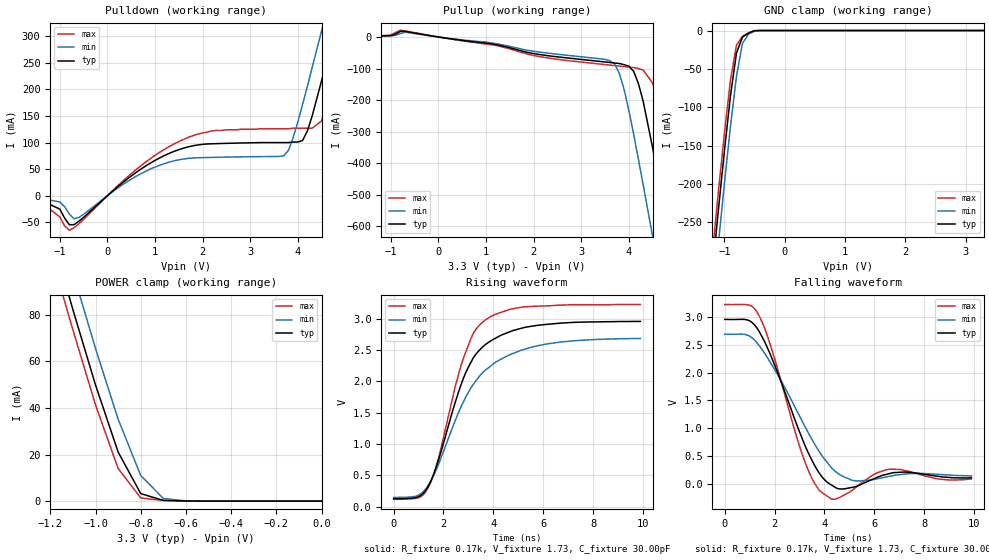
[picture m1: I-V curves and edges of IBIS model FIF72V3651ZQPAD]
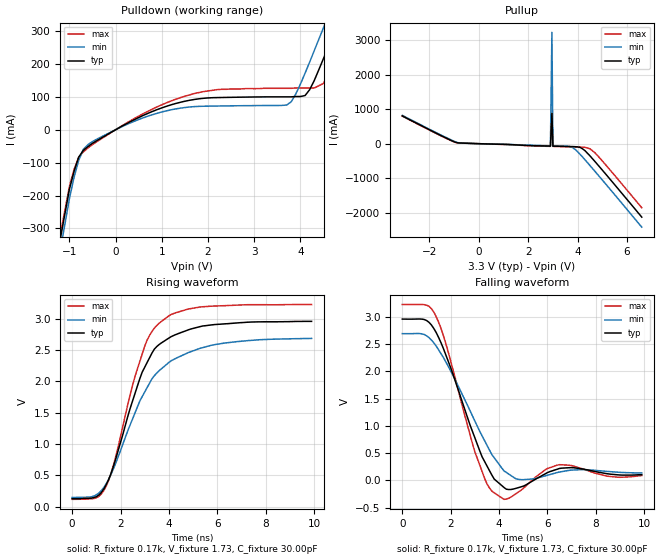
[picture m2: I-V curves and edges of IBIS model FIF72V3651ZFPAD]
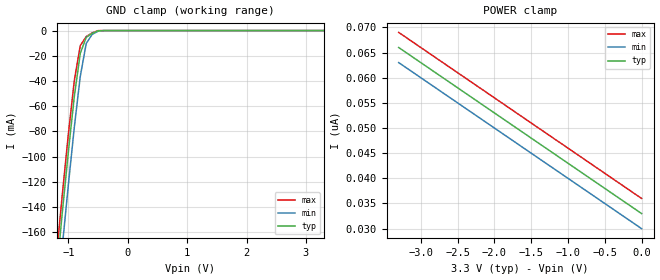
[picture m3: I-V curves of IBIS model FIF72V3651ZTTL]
| IBIS file i72v3641.ibs created by s2ibis2 version 1.1
| North Carolina State University Electronics Research Laboratory  1995
[IBIS ver]   2.1
[File name]   i72v3641.ibs
[File Rev]   1.0
[Date]   05/01/98
[Source]   Integrated Device Technology, Inc.
[Notes]   1. Temperatures: typ=25C, min=70C, max=0C 2. Cemos8_3.3v
   process. 3. Ramp rates based on 50 ohm load.
[Copyright]   Copyright 1997, Integrated Device Technology, Inc.
|   Component idt72V3641
[Component]   idt72V3641
[Manufacturer]   Integrated Device Technology
[Package]
| variable   typ   min   max
R_pkg   0.75   0.60   0.90
L_pkg   8.10nH   8.30nH   9.90nH
C_pkg   0.53pF   0.46pF   0.60pF
[Pin]  signal_name   model_name   R_pin   L_pin   C_pin
1   A35   FIF72V3651ZQPAD
2   A34   FIF72V3651ZQPAD
3   A33   FIF72V3651ZQPAD
4   A32   FIF72V3651ZQPAD
5   VCC   POWER
6   A31   FIF72V3651ZQPAD
7   A30   FIF72V3651ZQPAD
8   GND   GND
9   A29   FIF72V3651ZQPAD
10   A28   FIF72V3651ZQPAD
11   A27   FIF72V3651ZQPAD
12   A26   FIF72V3651ZQPAD
13   A25   FIF72V3651ZQPAD
14   A24   FIF72V3651ZQPAD
15   A23   FIF72V3651ZQPAD
16   GND   GND
17   A22   FIF72V3651ZQPAD
18   VCC   POWER
19   A21   FIF72V3651ZQPAD
20   A20   FIF72V3651ZQPAD
21   A19   FIF72V3651ZQPAD
22   A18   FIF72V3651ZQPAD
23   GND   GND
24   A17   FIF72V3651ZQPAD
25   A16   FIF72V3651ZQPAD
26   A15   FIF72V3651ZQPAD
27   A14   FIF72V3651ZQPAD
28   A13   FIF72V3651ZQPAD
29   VCC   POWER
30   A12   FIF72V3651ZQPAD
31   GND   GND
32   A11   FIF72V3651ZQPAD
33   A10   FIF72V3651ZQPAD
34   A9   FIF72V3651ZQPAD
35   A8   FIF72V3651ZQPAD
36   A7   FIF72V3651ZQPAD
37   A6   FIF72V3651ZQPAD
38   GND   GND
39   A5   FIF72V3651ZQPAD
40   A4   FIF72V3651ZQPAD
41   A3   FIF72V3651ZQPAD
42   VCC   POWER
43   A2   FIF72V3651ZQPAD
44   A1   FIF72V3651ZQPAD
45   A0   FIF72V3651ZQPAD
46   GND   GND
47   B0   FIF72V3651ZQPAD
48   B1   FIF72V3651ZQPAD
49   B2   FIF72V3651ZQPAD
50   B3   FIF72V3651ZQPAD
51   B4   FIF72V3651ZQPAD
52   A5   FIF72V3651ZQPAD
53   GND   GND
54   B6   FIF72V3651ZQPAD
55   VCC   POWER
56   B7   FIF72V3651ZQPAD
57   B8   FIF72V3651ZQPAD
58   B9   FIF72V3651ZQPAD
59   B10   FIF72V3651ZQPAD
60   B11   FIF72V3651ZQPAD
61   GND   GND
62   B12   FIF72V3651ZQPAD
63   B13   FIF72V3651ZQPAD
64   B14   FIF72V3651ZQPAD
65   B15   FIF72V3651ZQPAD
66   VCC   POWER
67   B16   FIF72V3651ZQPAD
68   B17   FIF72V3651ZQPAD
69   GND   GND
70   B18   FIF72V3651ZQPAD
71   B19   FIF72V3651ZQPAD
72   B20   FIF72V3651ZQPAD
73   B21   FIF72V3651ZQPAD
74   B22   FIF72V3651ZQPAD
75   B23   FIF72V3651ZQPAD
76   GND   GND
77   B24   FIF72V3651ZQPAD
78   B25   FIF72V3651ZQPAD
79   VCC   POWER
80   B26   FIF72V3651ZQPAD
81   B27   FIF72V3651ZQPAD
82   B28   FIF72V3651ZQPAD
83   B29   FIF72V3651ZQPAD
84   B30   FIF72V3651ZQPAD
85   B31   FIF72V3651ZQPAD
86   GND   GND
87   B32   FIF72V3651ZQPAD
88   B33   FIF72V3651ZQPAD
89   B34   FIF72V3651ZQPAD
90   B35   FIF72V3651ZQPAD
91   VCC   POWER
92   CLKB   FIF72V3651ZTTL
93   ENB   FIF72V3651ZTTL
94   WLRB   FIF72V3651ZTTL
95   CSBL   FIF72V3651ZTTL
96   GND   GND
97   MBF1L   FIF72V3651ZFPAD
98   GND   GND
99   MBB   FIF72V3651ZTTL
100   NC   NC
101   VCC   POWER
102   RFM   FIF72V3651ZTTL
103   RTM   FIF72V3651ZTTL
104   FS1SENL   FIF72V3651ZTTL
105   FS0SD   FIF72V3651ZTTL
106   GND   GND
107   RSTL   FIF72V3651ZTTL
108   MBA   FIF72V3651ZTTL
109   MBF2L   FIF72V3651ZFPAD
110   VCC   POWER
111   AEL   FIF72V3651ZFPAD
112   AFL   FIF72V3651ZFPAD
114   OR   FIF72V3651ZFPAD
115   IR   FIF72V3651ZFPAD
116   CSAL   FIF72V3651ZTTL
117   WRLA   FIF72V3651ZTTL
118   ENA   FIF72V3651ZTTL
119   CLKA   FIF72V3651ZTTL
120   GND   GND
| Models and submodels in the file (3): FIF72V3651ZQPAD (I/O), FIF72V3651ZFPAD (Output), FIF72V3651ZTTL (Input)
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| FIN  FIN   dummy_model
| QIN  QIN   dummy_model
| QOEL QOEL   dummy_model
|   Model FIF72V3651ZQPAD
[Model]   FIF72V3651ZQPAD
Model_type   I/O
Polarity   Non-Inverting
Enable   Active-Low
Vinl =  0.800V
Vinh =  2.000V
Vmeas =  1.500V
C_comp   3.00pF   NA   NA
[Temperature Range]   25.00   70.00   0.000
[Voltage Range]   3.30V   3.00V   3.60V
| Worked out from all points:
|   slope of the pulldown table from 0 to 0.495 V, typ, clamps not added: 13.5 ohm
|   slope of the pullup table from 0 to 0.495 V, typ, clamps not added: 46.5 ohm
|   GND clamp passes 1 mA (typ) near -0.52 V on its own axis
|   POWER clamp passes 1 mA (typ) near -0.72 V on its own axis
|   rising waveform, R_fixture 0.17k, V_fixture 1.73, C_fixture 30.00pF: 20-80 % time 1.47ns typ, 1.9ns min, 1.25ns max; typ from 0.128 V to 2.96 V
|   falling waveform, R_fixture 0.17k, V_fixture 1.73, C_fixture 30.00pF: 20-80 % time 1.46ns typ, 1.86ns min, 1.22ns max; typ from 2.96 V to 0.105 V
[Pulldown]
| voltage   I(typ)   I(min)   I(max)
-3.3V     -1mA       -1mA       -1mA
-1.5V     -4.2mA     -3.2mA     -5mA
-800mV    -54.6mA    -34.52mA   -64.94mA
-600mV    -47.99mA   -40.8mA    -52.81mA
600mV     43.67mA    36.44mA    48.95mA
1.5V      86.71mA    67.57mA    102mA
3.7V      100mA      75.02mA    126mA
4.1V      104mA      172mA      127mA
4.5V      217mA      311mA      141mA
4.7V      287mA      383mA      200mA
5.1V      430mA      528mA      340mA
6.6V      980mA      1.077A     888mA
[Pullup]
| voltage   I(typ)   I(min)   I(max)
-3.3V     300uA      300uA      300uA
-800mV    17.75mA    10.87mA    21.29mA
3.6V      -80.87mA   -75.44mA   -89.18mA
3.9V      -87.82mA   -167mA     -93.93mA
4.1V      -109mA     -309mA     -97.12mA
4.3V      -204mA     -469mA     -105mA
4.5V      -353mA     -634mA     -147mA
4.7V      -515mA     -801mA     -262mA
4.9V      -682mA     -970mA     -418mA
5.1V      -851mA     -1.14A     -583mA
5.3V      -1.02A     -1.31A     -751mA
6.6V      -2.136A    -2.428A    -1.864A
[GND_clamp]
| voltage   I(typ)   I(min)   I(max)
-3.3V     -2.102A    -2.142A    -2.08A
-1.2V     -314mA     -358mA     -291mA
-1.1V     -234mA     -278mA     -210mA
-1V       -157mA     -199mA     -134mA
-900mV    -85.1mA    -125mA     -64.47mA
-800mV    -29.4mA    -59.48mA   -19.05mA
-700mV    -8.491mA   -16.63mA   -7.437mA
-600mV    -3.454mA   -4.697mA   -2.961mA
-500mV    -293uA     -833uA     -94.53uA
-400mV    -15.41nA   -678nA     -4.678nA
3.3V      33nA       34.31nA    33nA
[POWER_clamp]
| voltage   I(typ)   I(min)   I(max)
-3.3V     879mA      893mA      871mA
-1.2V     116mA      132mA      107mA
-1.1V     82.2mA     98.22mA    73.49mA
-1V       49.87mA    65.51mA    41.33mA
-900mV    21.08mA    35.16mA    13.99mA
-800mV    3.228mA    11mA       1.36mA
-700mV    330uA      1.138mA    265uA
-600mV    63.58uA    105uA      57uA
0V        33nA       30nA       36nA
[Ramp]
| variable   typ   min   max
dV/dt_r   1.06/0.84n   0.90/0.96n   1.22/0.77n
dV/dt_f   1.54/1.40n   1.33/1.99n   1.73/1.11n
R_load = 50.00
[Rising Waveform]
R_fixture = 0.17k
V_fixture = 1.73
C_fixture = 30.00pF
R_dut = 0.75
L_dut = 8.10nH
C_dut = 0.53pF
| time   V(typ)   V(min)   V(max)
0s        128mV      147mV      118mV
1ns       159mV      186mV      143mV
1.4ns     338mV      348mV      314mV
1.8ns     744mV      677mV      775mV
2.8ns     2.051V     1.675V     2.373V
3.2ns     2.379V     1.956V     2.772V
3.6ns     2.561V     2.151V     2.956V
4.7ns     2.799V     2.433V     3.154V
5.7ns     2.891V     2.563V     3.201V
9.9ns     2.958V     2.686V     3.227V
[Falling Waveform]
R_fixture = 0.17k
V_fixture = 1.73
C_fixture = 30.00pF
R_dut = 0.75
L_dut = 8.10nH
C_dut = 0.53pF
| time   V(typ)   V(min)   V(max)
0s        2.959V     2.692V     3.227V
1ns       2.935V     2.659V     3.215V
1.4ns     2.729V     2.479V     3.009V
1.9ns     2.253V     2.136V     2.402V
3.1ns     823mV      1.134V     545mV
3.9ns     124mV      505mV      -158mV
4.4ns     -56.7mV    237mV      -280mV
5.2ns     -59.1mV    52.64mV    -89.82mV
6.6ns     181mV      132mV      260mV
9.9ns     105mV      140mV      85.54mV
|   Model FIF72V3651ZFPAD
[Model]   FIF72V3651ZFPAD
Model_type   Output
Vmeas =  1.500V
C_comp   3.00pF   NA   NA
[Temperature Range]   25.00   70.00   0.000
[Voltage Range]   3.30V   3.00V   3.60V
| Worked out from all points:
|   slope of the pulldown table from 0 to 0.495 V, typ, clamps not added: 13.5 ohm
|   slope of the pullup table from 0 to 0.495 V, typ, clamps not added: 46.5 ohm
|   rising waveform, R_fixture 0.17k, V_fixture 1.73, C_fixture 30.00pF: 20-80 % time 1.47ns typ, 1.86ns min, 1.28ns max; typ from 0.128 V to 2.96 V
|   falling waveform, R_fixture 0.17k, V_fixture 1.73, C_fixture 30.00pF: 20-80 % time 1.36ns typ, 1.7ns min, 1.14ns max; typ from 2.96 V to 0.104 V
[Pulldown]
| voltage   I(typ)   I(min)   I(max)
-3.3V     -2.095A    -2.135A    -2.074A
-1.5V     -565mA     -607mA     -542mA
-1V       -181mA     -210mA     -173mA
-700mV    -62.83mA   -59.84mA   -67.64mA
500mV     37.14mA    31.18mA    41.46mA
1.9V      95.58mA    71.46mA    116mA
3.7V      100mA      75.02mA    126mA
4.1V      104mA      172mA      127mA
4.5V      217mA      311mA      141mA
4.7V      287mA      383mA      200mA
5.1V      430mA      528mA      340mA
6.6V      980mA      1.077A     888mA
[Pullup]
| voltage   I(typ)   I(min)   I(max)
-3.1V     805mA      820mA      797mA
-1.5V     223mA      238mA      214mA
-1V       54.39mA    68.64mA    47.35mA
-800mV    20.98mA    21.87mA    22.65mA
2.9V      -69.66mA   -61.22mA   -77.9mA
2.96V     879mA      3.227A     871mA
3V        -71.29mA   -62.83mA   -79.53mA
3.8V      -84.18mA   -116mA     -92.35mA
4.1V      -108mA     -308mA     -97.12mA
4.5V      -352mA     -632mA     -147mA
4.9V      -680mA     -967mA     -417mA
6.6V      -2.129A    -2.419A    -1.857A
[Ramp]
| variable   typ   min   max
dV/dt_r   1.06/0.84n   0.90/0.98n   1.22/0.78n
dV/dt_f   1.54/1.26n   1.34/1.63n   1.73/1.06n
R_load = 50.00
[Rising Waveform]
R_fixture = 0.17k
V_fixture = 1.73
C_fixture = 30.00pF
R_dut = 0.75
L_dut = 8.10nH
C_dut = 0.53pF
| time   V(typ)   V(min)   V(max)
0s        128mV      147mV      118mV
1ns       160mV      189mV      143mV
1.4ns     344mV      360mV      321mV
1.7ns     634mV      598mV      651mV
2.5ns     1.69V      1.403V     1.941V
3ns       2.226V     1.831V     2.562V
3.6ns     2.59V      2.172V     2.93V
4.3ns     2.75V      2.371V     3.098V
5.8ns     2.904V     2.581V     3.202V
9.9ns     2.959V     2.687V     3.227V
[Falling Waveform]
R_fixture = 0.17k
V_fixture = 1.73
C_fixture = 30.00pF
R_dut = 0.75
L_dut = 8.10nH
C_dut = 0.53pF
| time   V(typ)   V(min)   V(max)
0s        2.959V     2.692V     3.227V
900ps     2.952V     2.677V     3.224V
1.4ns     2.713V     2.464V     3.003V
1.8ns     2.3V       2.173V     2.508V
3ns       779mV      1.087V     522mV
3.5ns     263mV      643mV      -66.12mV
3.8ns     21.74mV    413mV      -231mV
4.7ns     -148mV     25.59mV    -246mV
6.5ns     217mV      152mV      286mV
9.9ns     104mV      136mV      87.61mV
|   Model FIF72V3651ZTTL
[Model]   FIF72V3651ZTTL
Model_type   Input
Vinl =  0.800V
Vinh =  2.000V
Vmeas =  1.400V
C_comp   3.00pF   NA   NA
[Temperature Range]   25.00   70.00   0.000
[Voltage Range]   3.30V   3.00V   3.60V
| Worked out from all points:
|   GND clamp passes 1 mA (typ) near -0.54 V on its own axis
[GND_clamp]
| voltage   I(typ)   I(min)   I(max)
-3.3V     -1.289A    -1.313A    -1.275A
-1.2V     -193mA     -219mA     -178mA
-1.1V     -143mA     -170mA     -129mA
-1V       -95.93mA   -122mA     -81.79mA
-900mV    -52.03mA   -76.45mA   -39.47mA
-800mV    -18.07mA   -36.3mA    -11.9mA
-700mV    -5.417mA   -10.25mA   -4.762mA
-600mV    -2.198mA   -2.995mA   -1.861mA
-500mV    -168uA     -522uA     -41.7uA
-400mV    -10.73nA   -401nA     -4.4nA
3.3V      33nA       33nA       33nA
[POWER_clamp]
| voltage   I(typ)   I(min)   I(max)
-3.3V     66nA       63nA       69nA
-3.2V     65nA       62nA       68nA
-3V       63nA       60nA       66nA
0V        33nA       30nA       36nA
